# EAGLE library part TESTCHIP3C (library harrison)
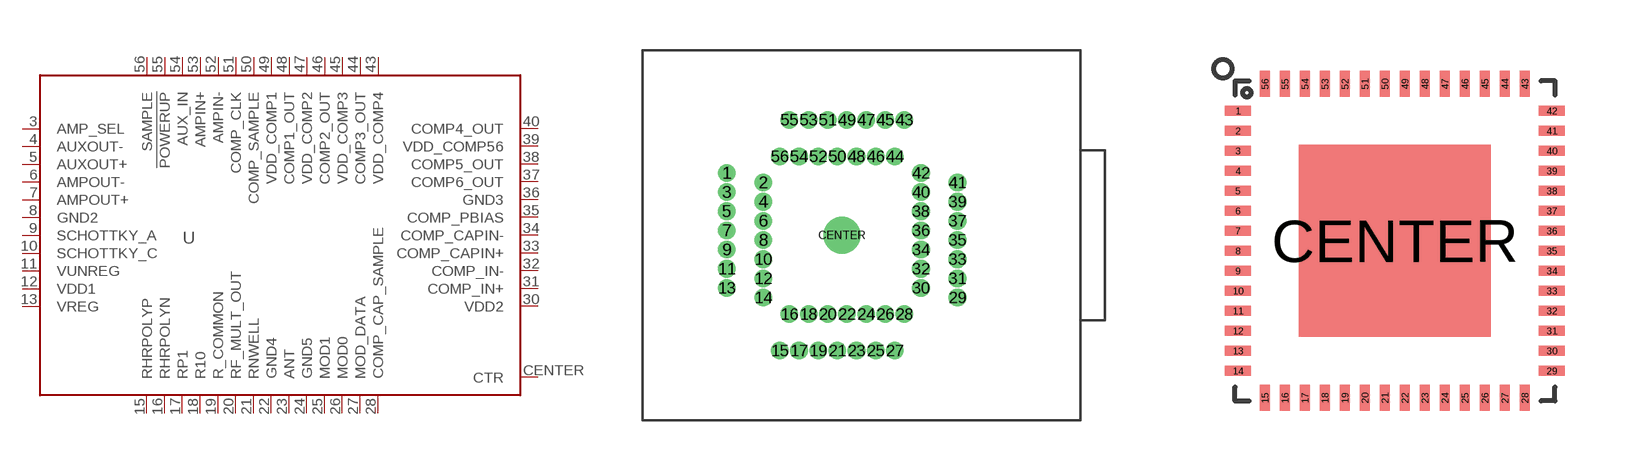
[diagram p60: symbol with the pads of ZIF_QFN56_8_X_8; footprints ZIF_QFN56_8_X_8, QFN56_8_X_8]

Designator prefix U

## TESTCHIP3C_ZIF  [ZIF_QFN56_8_X_8]
3  AMP_SEL  in
4  AUXOUT-  out
5  AUXOUT+  out
6  AMPOUT-  out
7  AMPOUT+  out
8  GND2  pwr
9  SCHOTTKY_A  pas
10  SCHOTTKY_C  pas
11  VUNREG  pwr
12  VDD1  pwr
13  VREG  pwr
15  RHRPOLYP  pas
16  RHRPOLYN  pas
17  RP1  pas
18  R10  pas
19  R_COMMON  pas
20  RF_MULT_OUT  pas
21  RNWELL  pas
22  GND4  pwr
23  ANT  pas
24  GND5  pwr
25  MOD1  in
26  MOD0  in
27  MOD_DATA  in
28  COMP_CAP_SAMPLE  in
30  VDD2  pwr
31  COMP_IN+  in
32  COMP_IN-  in
33  COMP_CAPIN+  in
34  COMP_CAPIN-  in
35  COMP_PBIAS  in
36  GND3  pwr
37  COMP6_OUT  out
38  COMP5_OUT  out
39  VDD_COMP56  pwr
40  COMP4_OUT  out
43  VDD_COMP4  pwr
44  COMP3_OUT  out
45  VDD_COMP3  pwr
46  COMP2_OUT  out
47  VDD_COMP2  pwr
48  COMP1_OUT  out
49  VDD_COMP1  pwr
50  COMP_SAMPLE  in
51  COMP_CLK  in
52  AMPIN-  in
53  AMPIN+  in
54  AUX_IN  in
55  !POWERUP!  in
56  SAMPLE  in
CENTER  CTR  pwr

## TESTCHIP3C_QFN  [QFN56_8_X_8]
Pads as for ZIF_QFN56_8_X_8

## Footprint ZIF_QFN56_8_X_8 (pad centres in mm)
drill 0.41 pad 0.813: 1 -6.02,3.251; 2 -4.115,2.751; 3 -6.02,2.25; 4 -4.115,1.75; 5 -6.02,1.25; 6 -4.115,0.752; 7 -6.02,0.249; 8 -4.115,-0.249; 9 -6.02,-0.749; 10 -4.115,-1.25; 11 -6.02,-1.75; 12 -4.115,-2.25; 13 -6.02,-2.751; 14 -4.115,-3.251; 15 -3.251,-6.02; 16 -2.751,-4.115; 17 -2.25,-6.02; 18 -1.75,-4.115; 19 -1.25,-6.02; 20 -0.752,-4.115; 21 -0.249,-6.02; 22 0.249,-4.115; 23 0.749,-6.02; 24 1.25,-4.115; 25 1.75,-6.02; 26 2.25,-4.115; 27 2.751,-6.02; 28 3.251,-4.115; 29 6.02,-3.251; 30 4.115,-2.751; 31 6.02,-2.25; 32 4.115,-1.75; 33 6.02,-1.25; 34 4.115,-0.752; 35 6.02,-0.249; 36 4.115,0.249; 37 6.02,0.749; 38 4.115,1.25; 39 6.02,1.75; 40 4.115,2.25; 41 6.02,2.751; 42 4.115,3.251; 43 3.251,6.02; 44 2.751,4.115; 45 2.25,6.02; 46 1.75,4.115; 47 1.25,6.02; 48 0.752,4.115; 49 0.249,6.02; 50 -0.249,4.115; 51 -0.749,6.02; 52 -1.25,4.115; 53 -1.75,6.02; 54 -2.25,4.115; 55 -2.751,6.02; 56 -3.251,4.115
drill 1.02 pad 1.93: CENTER 0,0

## Footprint QFN56_8_X_8 (pad centres in mm)
smd 0.65 x 0.25: 1 -3.925,3.25; 2 -3.925,2.75; 3 -3.925,2.25; 4 -3.925,1.75; 5 -3.925,1.25; 6 -3.925,0.75; 7 -3.925,0.25; 8 -3.925,-0.25; 9 -3.925,-0.75; 10 -3.925,-1.25; 11 -3.925,-1.75; 12 -3.925,-2.25; 13 -3.925,-2.75; 14 -3.925,-3.25; 29 3.925,-3.25; 30 3.925,-2.75; 31 3.925,-2.25; 32 3.925,-1.75; 33 3.925,-1.25; 34 3.925,-0.75; 35 3.925,-0.25; 36 3.925,0.25; 37 3.925,0.75; 38 3.925,1.25; 39 3.925,1.75; 40 3.925,2.25; 41 3.925,2.75; 42 3.925,3.25
smd 0.25 x 0.65: 15 -3.25,-3.925; 16 -2.75,-3.925; 17 -2.25,-3.925; 18 -1.75,-3.925; 19 -1.25,-3.925; 20 -0.75,-3.925; 21 -0.25,-3.925; 22 0.25,-3.925; 23 0.75,-3.925; 24 1.25,-3.925; 25 1.75,-3.925; 26 2.25,-3.925; 27 2.75,-3.925; 28 3.25,-3.925; 43 3.25,3.925; 44 2.75,3.925; 45 2.25,3.925; 46 1.75,3.925; 47 1.25,3.925; 48 0.75,3.925; 49 0.25,3.925; 50 -0.25,3.925; 51 -0.75,3.925; 52 -1.25,3.925; 53 -1.75,3.925; 54 -2.25,3.925; 55 -2.75,3.925; 56 -3.25,3.925
smd 4.8 x 4.8: CENTER 0,0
